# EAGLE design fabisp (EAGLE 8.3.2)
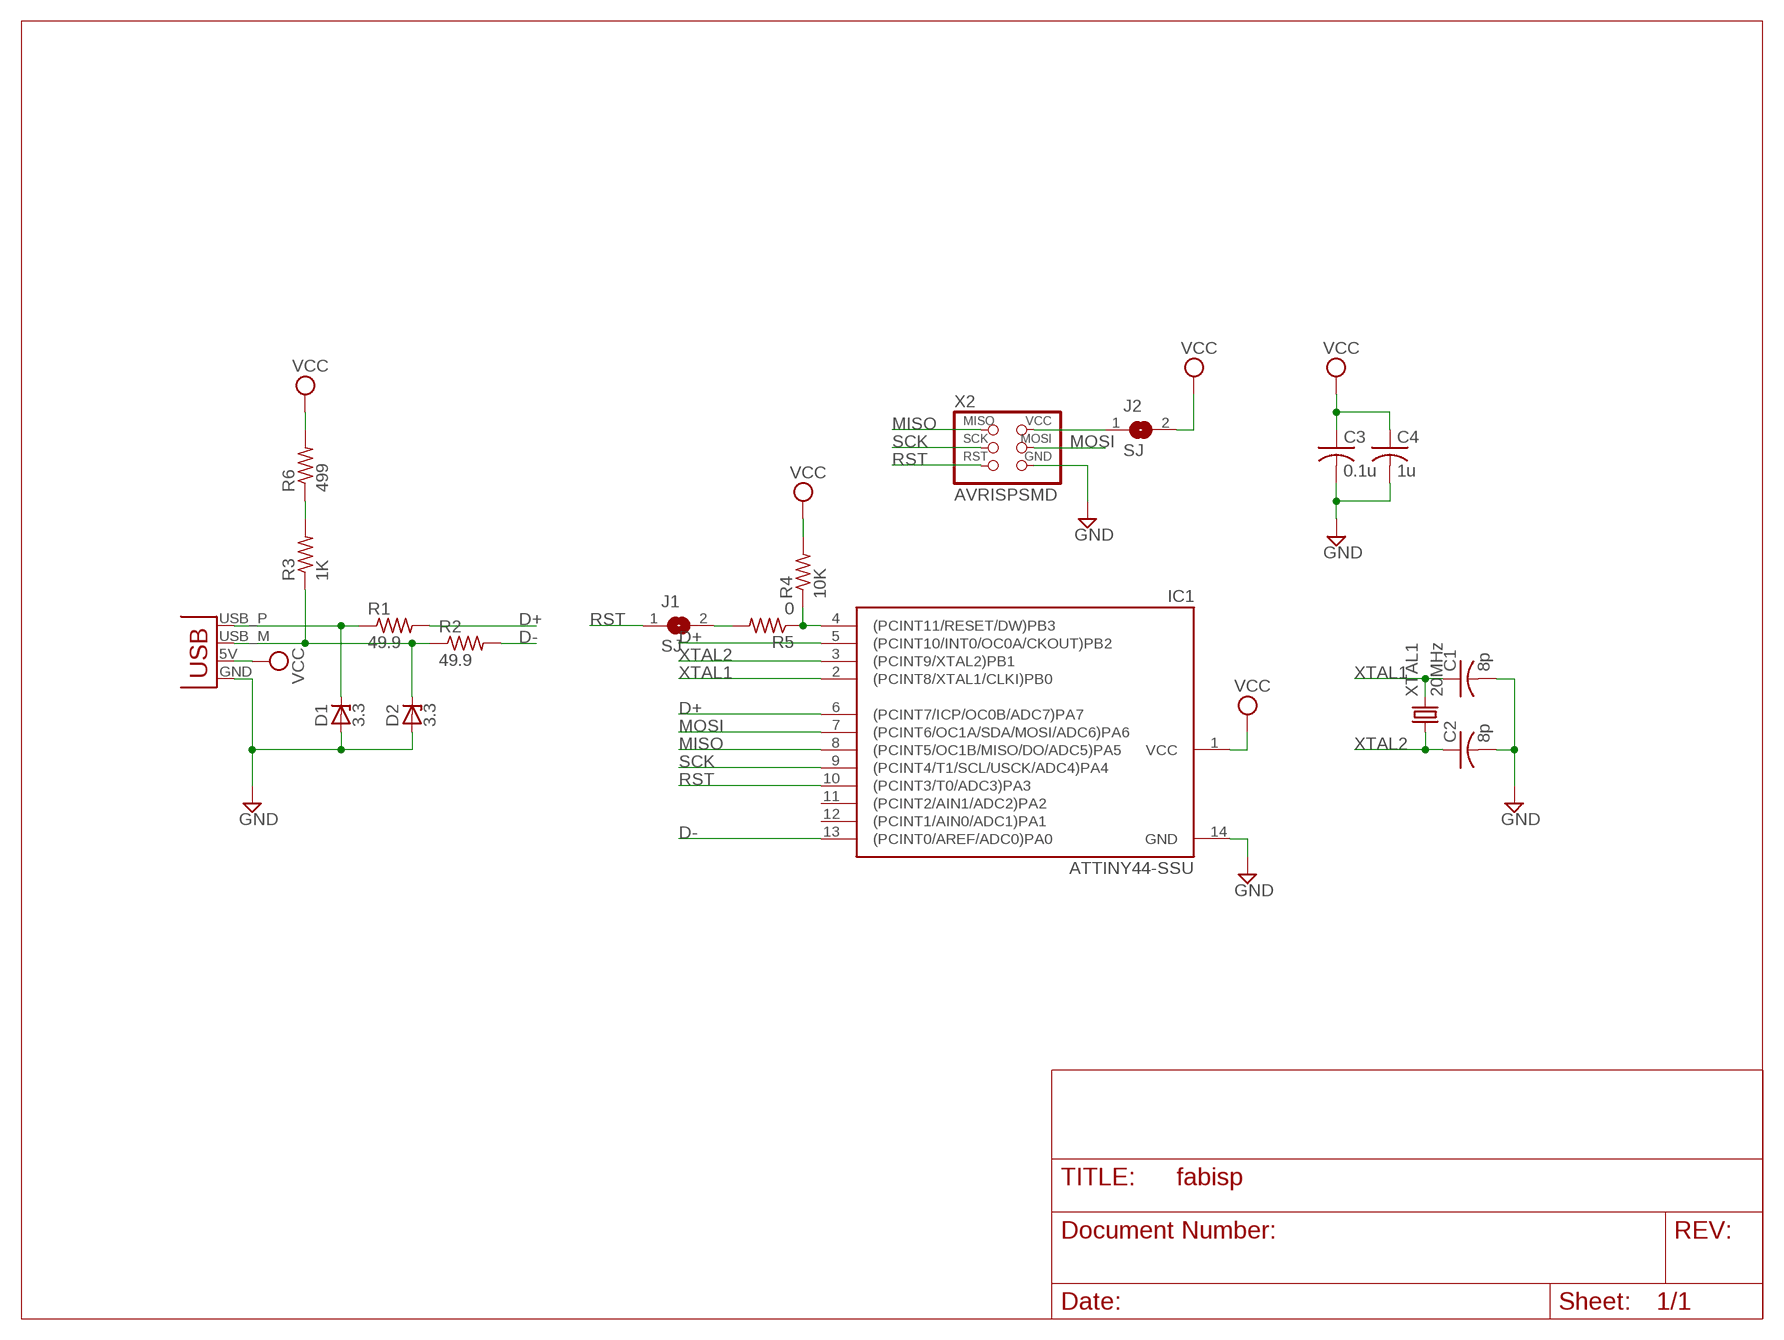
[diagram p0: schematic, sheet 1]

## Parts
C1  8p  C-USC1206  [C1206]
C2  8p  C-USC1206  [C1206]
C3  0.1u  C-USC1206  [C1206]
C4  1u  C-USC1206  [C1206]
D1  3.3  ZENER_DIODESOD123  [SOD123]
D2  3.3  ZENER_DIODESOD123  [SOD123]
IC1  ATTINY44-SSU  [SOIC14]
J1  SJ  SOLDER_JUMPER  [SJFAB]
J2  SJ  SOLDER_JUMPER  [SJFAB]
R1  49.9  R-US_R1206  [R1206]
R2  49.9  R-US_R1206  [R1206]
R3  1K  R-US_R1206  [R1206]
R4  10K  R-US_R1206  [R1206]
R5  0  R-US_R1206  [R1206]
R6  499  R-US_R1206  [R1206]
X1  USBPCB  [USB-A-PCB]
X2  AVRISPSMD  [2X03SMD]
XTAL1  20MHz  CSM-7X-DU  [CSM-7X-DU]

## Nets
D+: IC1.5((PCINT10/INT0/OC0A/CKOUT)PB2) IC1.6((PCINT7/ICP/OC0B/ADC7)PA7) R1.2
D-: IC1.13((PCINT0/AREF/ADC0)PA0) R2.2
GND: C1.2 C2.2 C3.2 C4.2 D1.ANODE D2.ANODE IC1.14(GND) X1.GND X2.6(GND)
MISO: IC1.8((PCINT5/OC1B/MISO/DO/ADC5)PA5) X2.1(MISO)
MOSI: IC1.7((PCINT6/OC1A/SDA/MOSI/ADC6)PA6) X2.4(MOSI)
N$1: D1.CATHODE R1.1 X1.USB_P(D+)
N$2: D2.CATHODE R2.1 R3.1 X1.USB_M(D-)
N$3: J1.2 R5.2
N$4: J2.1 X2.2(VCC)
N$5: IC1.4((PCINT11/RESET/DW)PB3) R4.1 R5.1
N$6: R3.2 R6.1
RST: IC1.10((PCINT3/T0/ADC3)PA3) J1.1 X2.5(RST)
SCK: IC1.9((PCINT4/T1/SCL/USCK/ADC4)PA4) X2.3(SCK)
VCC: C3.1 C4.1 IC1.1(VCC) J2.2 R4.2 R6.2 X1.5V(VBUS)
XTAL1: C1.1 IC1.2((PCINT8/XTAL1/CLKI)PB0) XTAL1.2
XTAL2: C2.1 IC1.3((PCINT9/XTAL2)PB1) XTAL1.1
Unconnected: IC1.11((PCINT2/AIN1/ADC2)PA2) IC1.12((PCINT1/AIN0/ADC1)PA1)

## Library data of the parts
C1-C4 = rcl:C-US: CAPACITOR, American symbol
D1 D2 = fab:ZENER_DIODE: zener diode
IC1 = fab:ATTINY44
J1 J2 = fab:SOLDER_JUMPER
R1-R6 = rcl:R-US_: RESISTOR, American symbol
X1 = SparkFun:USB: USB Connectors USB-B-PTH is fully proven SKU : PRT-00139 USB-miniB is fully proven SKU : PRT-00587 USB-A-PCB is untested. USB-A-H is throughly reviewed, but untested. Spark Fun Electronics SKU : PRT-00437 USB-B-SMT is throughly reviewed, but untested. Needs silkscreen touching up. USB-A-S has not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
X2 = fab:AVRISP
XTAL1 = crystal:CSM-7X-DU: SMD CRYSTAL; OC_FARNELL: unknown; OC_NEWARK: unknown

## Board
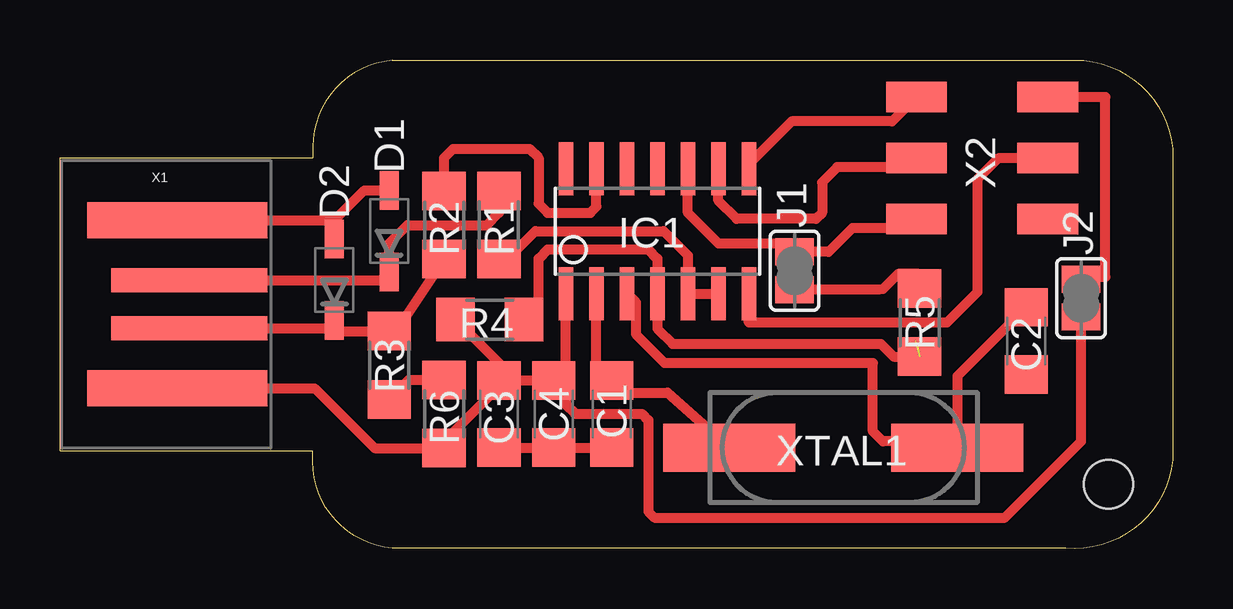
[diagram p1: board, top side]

Size 46.35 x 20.36 mm. Coordinates in mm from the lower left corner, seen from the top.
Outline: 0,4.08 10.54,4.08 10.54,3.95 arc90 13.84,0.02 41.91,0.02 arc90 46.35,3.7 46.35,16.65 arc90 41.91,20.34 13.84,20.34 arc90 10.54,16.4 10.54,16.27 0,16.27 0,4.08
Copper layers (1*16): Top 0.035mm / dielectric 1.5mm / Bottom 0.035mm
Design rules "fab": minimum track width 12mil, minimum drill 0.8mm, track to track 15.5mil, track to pad 15.5mil, pad to pad 15mil, via to via 15mil, smd to smd 10mil, copper to edge 0mil, drill to drill 1mm, minimum pad ring 0.2mm, minimum via ring 0.2mm, stop-mask expansion 4mil, vias tented up to drill 0mil, thermal gap 1mm
Holes 2.03 mm at 43.69,2.68
tRestrict: 4 lines

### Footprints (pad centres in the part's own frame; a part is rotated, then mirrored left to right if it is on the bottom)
C1206 = smd 1.6 x 1.8: 1 -1.4,0; 2 1.4,0
SOD123 = smd 1.6 x 0.8: ANODE 1.7,0; CATHODE -1.7,0
SOIC14 = smd 0.61 x 2.21: 1 -3.81,-2.603; 2 -2.54,-2.603; 3 -1.27,-2.603; 4 0,-2.603; 5 1.27,-2.603; 6 2.54,-2.603; 7 3.81,-2.603; 8 3.81,2.603; 9 2.54,2.603; 10 1.27,2.603; 11 0,2.603; 12 -1.27,2.603; 13 -2.54,2.603; 14 -3.81,2.603
SJFAB = smd 1.118 x 1.6: 1 -0.787,0; 2 0.787,0
R1206 = smd 1.6 x 1.803: 1 -1.422,0; 2 1.422,0
USB-A-PCB = smd 7.5 x 1.5: 5V -0.2,-3.5; GND -0.2,3.5 | smd 6.5 x 1: USB_M 0.3,-1; USB_P 0.3,1
2X03SMD = smd 2.54 x 1.27: 1 -2.54,2.54; 2 2.92,2.54; 3 -2.54,0; 4 2.92,0; 5 -2.54,-2.54; 6 2.92,-2.54
CSM-7X-DU = smd 5.5 x 2: 1 -4.75,0; 2 4.75,0

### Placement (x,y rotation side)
C1  22.99,5.61 270 top
C2  40.26,8.65 270 top
C3  18.29,5.61 270 top
C4  20.57,5.61 270 top
D1  13.72,13.23 90 top
D2  11.43,11.19 90 top
IC1  24.89,13.23 0 top
J1  30.61,11.57 270 top
J2  42.55,10.43 270 top
R1  18.29,13.48 270 top
R2  16,13.48 90 top
R3  13.72,7.64 270 top
R4  17.91,9.54 180 top
R5  35.81,9.42 90 top
R6  16,5.61 270 top
X1  5.08,10.18 0 top
X2  38.23,16.27 0 top
XTAL1  32.64,4.21 180 top

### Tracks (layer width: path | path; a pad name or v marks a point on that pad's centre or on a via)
D+
  Top 0.406: IC1.6 IC1.5 26.16,12.21 25.15,13.23 19.81,13.23 18.64,12.06 R1.2
D-
  Top 0.406: IC1.13 22.35,14.24 22.1,13.99 20.32,13.99 19.94,14.37 19.94,16.27 19.56,16.65 16.38,16.65 16,16.27 R2.2
GND
  Top 0.406: X1.GND 11.43,13.68 | 11.43,13.68 D2.ANODE | D1.ANODE 12.68,14.93 11.43,13.68 | C1.2 C4.2 C3.2
MISO
  Top 0.406: 28.7,15.89 28.7,16.27 | 28.7,15.89 IC1.8 | X2.1 34.67,17.8 30.48,17.8 28.7,16.02 28.7,15.89
MOSI
  Top 0.406: 28.7,10.43 IC1.7 28.7,9.42 36.96,9.42 38.23,10.69 38.23,15.38 39.12,16.27 X2.4
N$1
  Top 0.406: D1.CATHODE 13.56,11.69 | X1.USB_P 13.37,11.18 D1.CATHODE | R1.1 18.29,13.99 17.78,13.48 14.48,13.48 13.72,12.72 D1.CATHODE
N$2
  Top 0.406: X1.USB_M 11.11,9.18 D2.CATHODE 11.43,9.06 R3.1 14.02,9.06 R2.1
N$3
  Top 0.406: J1.2 31.11,10.79 31.14,10.79 34.13,10.79 34.28,10.81 34.92,11.45 35.79,11.45 R5.2
N$4
  Top 0.406: 42.82,11.22 J2.1 42.55,11.32 43.56,11.32 43.56,18.81 X2.2
N$5  (2 unrouted)
  Top 0.305: R4.1 19.94,10.15
  Top 0.406: 19.94,10.15 19.94,12.08 20.32,12.46 24.51,12.46 24.89,12.08 IC1.4 24.89,9.16 25.53,8.53 34.2,8.53 34.74,7.99 R5.1
N$6
  Top 0.406: R6.1 14.53,7.03 R3.2
RST
  Top 0.406: IC1.10 26.16,13.99 27.43,12.72 30,12.72 J1.1 32.03,12.36 33.02,13.35 35.31,13.35 X2.5 34.8,13.73
SCK
  Top 0.406: IC1.9 27.43,14.5 28.19,13.73 31.5,13.73 31.75,13.99 31.75,15.26 32.38,15.89 35.31,15.89 X2.3
VCC
  Top 0.406: 21.08,7.51 IC1.1 | 21.08,7.51 C4.1 C3.1 | X1.5V 10.61,6.68 13.11,4.18 R6.2 16,4.46 17.91,6.37 17.91,6.62 C3.1 | R4.2 18.29,7.74 C3.1 | 21.08,7.51 21.08,5.99 21.46,5.61 24.26,5.61 24.51,5.35 24.51,1.54 24.77,1.29 39.37,1.29 42.55,4.46 J2.2
XTAL1
  Top 0.406: IC1.2 22.35,7.64 C1.1 23.24,7.01 23.75,6.49 25.3,6.49 XTAL1.2
XTAL2
  Top 0.406: C2.1 37.39,7.18 XTAL1.1 37.13,4.46 34.29,4.46 33.87,4.88 33.87,7.73 25.2,7.73 23.99,8.93 23.99,10.25 IC1.3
